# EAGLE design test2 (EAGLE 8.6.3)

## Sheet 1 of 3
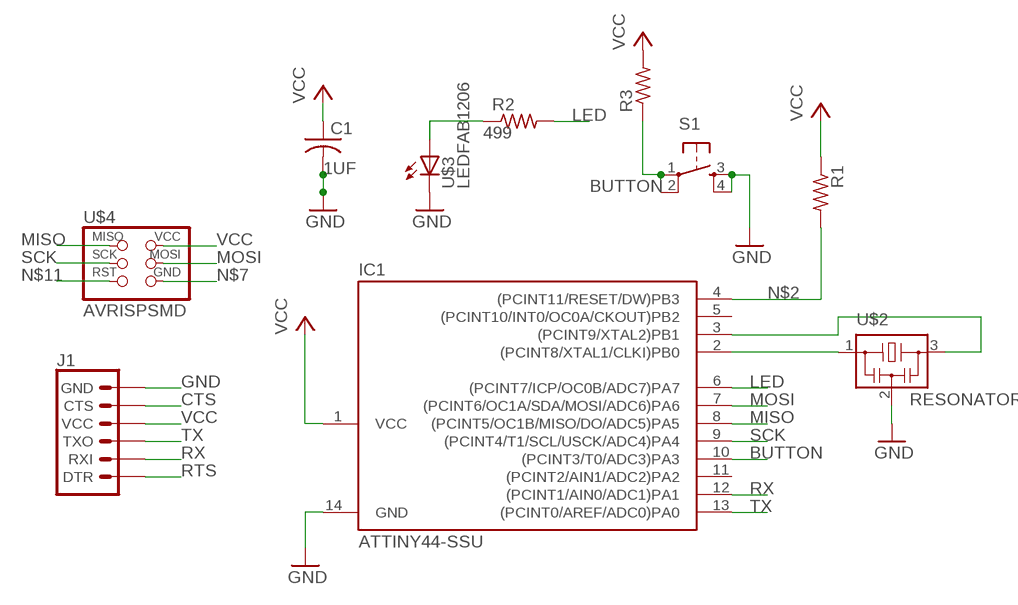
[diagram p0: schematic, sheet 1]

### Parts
C1  C-USC1210  [C1210]
IC1  ATTINY44-SSU  [SOIC14]
J1  6_PIN_SERIAL_TARGETSMD  [1X06-SMD_RA_MALE]
R1  RES-US1206FAB  [R1206FAB]
R2  RES-US1206FAB  [R1206FAB]
R3  RES-US1206FAB  [R1206FAB]
S1  6MM_SWITCH6MM_SWITCH  [6MM_SWITCH]
U$2  RESONATOR  [EFOBM]
U$3  LEDFAB1206  [LED1206FAB]
U$4  AVRISPSMD  [2X03SMD]

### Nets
1UF: C1.2 ; supply symbol labelled GND
499: R2.1 U$3.1(A)
BUTTON: IC1.10((PCINT3/T0/ADC3)PA3) R3.1 S1.1(P) S1.2(P1)
CTS: J1.5(CTS)
GND: J1.6(GND)
LED: IC1.6((PCINT7/ICP/OC0B/ADC7)PA7) R2.2
MISO: IC1.8((PCINT5/OC1B/MISO/DO/ADC5)PA5) U$4.1(MISO)
MOSI: IC1.7((PCINT6/OC1A/SDA/MOSI/ADC6)PA6) U$4.4(MOSI)
N$2: IC1.4((PCINT11/RESET/DW)PB3) R1.2
N$4: IC1.3((PCINT9/XTAL2)PB1) U$2.3
N$7: IC1.14(GND) S1.3(S) S1.4(S1) U$2.2 U$3.2(C) U$4.6(GND) ; supply symbol labelled GND
N$11: U$4.5(RST)
N$23: IC1.2((PCINT8/XTAL1/CLKI)PB0) U$2.1
RTS: J1.1(DTR)
RX: IC1.12((PCINT1/AIN0/ADC1)PA1) J1.2(RXI)
SCK: IC1.9((PCINT4/T1/SCL/USCK/ADC4)PA4) U$4.3(SCK)
TX: IC1.13((PCINT0/AREF/ADC0)PA0) J1.3(TXO)
VCC: C1.1 IC1.1(VCC) J1.4(VCC) R1.1 R3.2 U$4.2(VCC)
Unconnected: IC1.5((PCINT10/INT0/OC0A/CKOUT)PB2) IC1.11((PCINT2/AIN1/ADC2)PA2)

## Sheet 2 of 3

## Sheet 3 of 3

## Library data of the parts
C1 = rcl:C-US: CAPACITOR, American symbol; SPICEPREFIX: C
IC1 = fab:ATTINY44
J1 = SparkFun-Connectors:6_PIN_SERIAL_TARGET: 6-pin header connection for use with the "FTDI BASIC" pinout - TARGET SIDE. Also known as "Arduino Serial Program Header". It is used to mate with our FTDI Basic serial programmers using the Arduino IDE. Note, this device has "TARGET" in the name. It is intended to be used on a design that contains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; PROD_ID: CONN-08971
R1-R3 = fab:RES-US: Resistor (US Symbol)
S1 = fab:6MM_SWITCH: OMRON SWITCH
U$2 = fab:RESONATOR
U$3 = fab:LED: LED
U$4 = fab:AVRISP

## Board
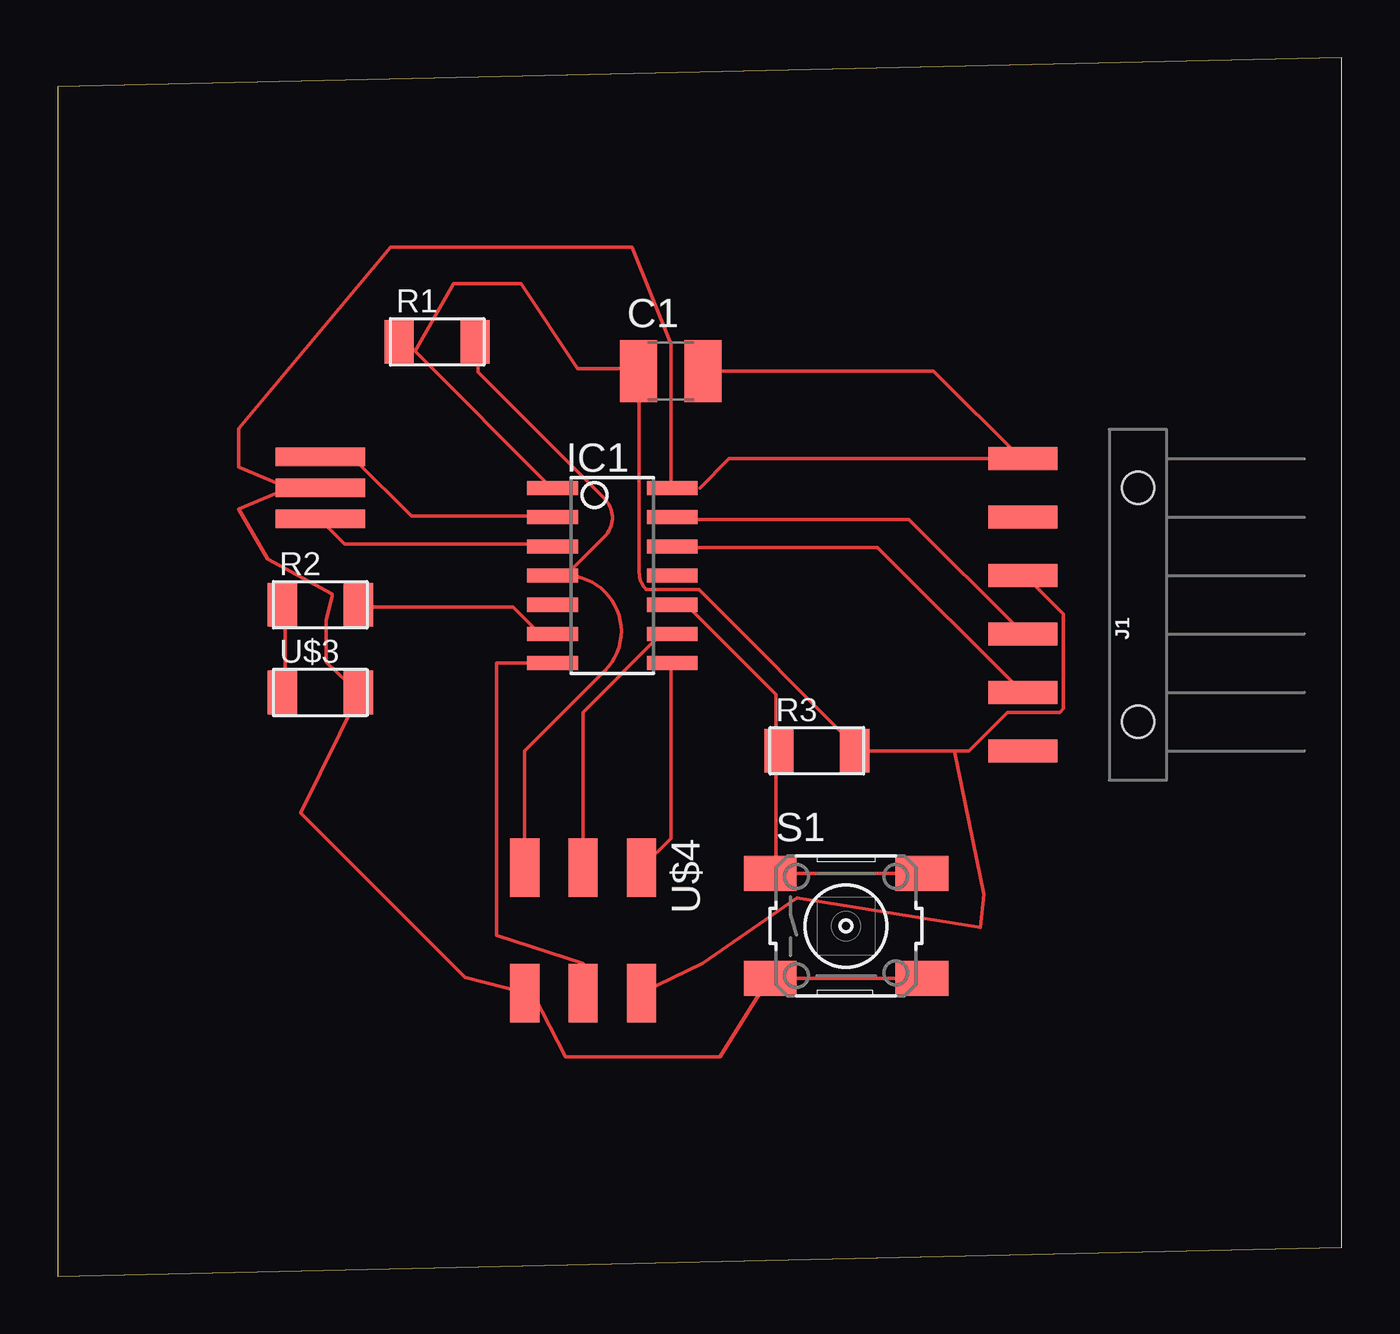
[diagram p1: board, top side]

Size 55.86 x 53.01 mm. Coordinates in mm from the lower left corner, seen from the top.
Outline: 0,0 55.86,1.27 55.86,53.01 0,51.74 0,0
Copper layers (1*16): Top 0.035mm / dielectric 1.5mm / Bottom 0.035mm
Design rules "default": minimum track width 6mil, minimum drill 0.35mm, track to track 6mil, track to pad 6mil, pad to pad 6mil, via to via 6mil, smd to smd 6mil, copper to edge 40mil, drill to drill 6mil, minimum pad ring 10mil, minimum via ring 8mil, stop-mask expansion 4mil, vias tented up to drill 0mil, thermal gap 10mil

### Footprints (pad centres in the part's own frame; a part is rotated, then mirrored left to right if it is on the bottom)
C1210 = smd 1.6 x 2.7: 1 -1.4,0; 2 1.4,0
SOIC14 = smd 0.61 x 2.21: 1 -3.81,-2.603; 2 -2.54,-2.603; 3 -1.27,-2.603; 4 0,-2.603; 5 1.27,-2.603; 6 2.54,-2.603; 7 3.81,-2.603; 8 3.81,2.603; 9 2.54,2.603; 10 1.27,2.603; 11 0,2.603; 12 -1.27,2.603; 13 -2.54,2.603; 14 -3.81,2.603
1X06-SMD_RA_MALE = smd 1 x 3: 1 -6.35,5; 2 -3.81,5; 3 -1.27,5; 4 1.27,5; 5 3.81,5; 6 6.35,5 | hole 1.4: -5.08,0; 5.08,0
R1206FAB = smd 1.27 x 1.905: 1 -1.651,0; 2 1.651,0
6MM_SWITCH = smd 2.286 x 1.524: 1 -3.302,2.286; 2 3.302,2.286; 3 -3.302,-2.286; 4 3.302,-2.286
EFOBM = smd 0.8 x 3.9: 1 -1.35,0; 2 0,0; 3 1.35,0
LED1206FAB = smd 1.27 x 1.905: 1 -1.651,0; 2 1.651,0
2X03SMD = smd 2.54 x 1.27: 1 -2.54,2.54; 2 2.92,2.54; 3 -2.54,0; 4 2.92,0; 5 -2.54,-2.54; 6 2.92,-2.54

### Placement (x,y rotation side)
C1  26.67,39.37 0 top
IC1  24.13,30.48 270 top
J1  46.99,29.21 90 top
R1  16.51,40.64 0 top
R2  11.43,29.21 0 top
R3  33.02,22.86 0 top
S1  34.29,15.24 0 top
U$2  11.43,34.29 270 top
U$3  11.43,25.4 0 top
U$4  22.86,15.24 270 top

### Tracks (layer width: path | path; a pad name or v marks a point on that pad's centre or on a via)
499
  Top 0.152: U$3.1 9.91,25.45 9.91,29.11 R2.1
BUTTON
  Top 0.152: 31.24,22.86 31.24,17.68 31.09,17.53 | 31.24,22.86 31.24,25.3 27.43,29.11 26.82,29.11 IC1.10 | 31.24,22.86 R3.1 | 31.09,17.53 S1.2 | 31.09,17.53 S1.1
LED
  Top 0.152: R2.2 13.11,29.11 19.81,29.11 20.88,28.04 21.49,28.04 IC1.6
MISO
  Top 0.152: U$4.1 26.67,19.05 26.67,26.67 IC1.8
MOSI
  Top 0.152: IC1.7 19.1,26.67 19.1,14.83 22.86,13.61 U$4.4
N$1
  Top 0.152: 27.94,39.37 38.1,39.37 41.91,35.56
N$2
  Top 0.152: 22.1,30.48 arc-135 23.81,26.35 20.32,22.86 20.32,19.05 | 22.1,30.48 23.79,32.17 arc90 23.79,33.82 18.29,39.32 18.29,40.54 R1.2 | IC1.4 21.59,30.48 22.1,30.48
N$3
  Top 0.152: 27.94,34.29 29.21,35.56 40.64,35.56
N$4
  Top 0.152: IC1.3 21.49,31.85 12.5,31.85 11.43,32.92 U$2.3
N$7
  Top 0.152: S1.4 S1.3 30.94,12.95 28.8,9.55 22.1,9.55 20.73,12.19 20.42,12.19 U$4.6 20.27,12.34 17.73,13.01 10.57,20.17 13.11,25.3 U$3.2 11.68,26.72 11.68,28.55 11.94,29.57 11.94,29.67 9.14,31.19 7.87,33.38 10.06,34.29 | 10.06,34.29 7.87,35.2 7.87,36.88 14.48,44.76 24.99,44.76 26.67,40.54 26.67,34.29 IC1.14 | 10.06,34.29 U$2.2
N$23
  Top 0.152: IC1.2 21.49,33.07 15.39,33.07 12.95,35.51 11.43,35.51 U$2.1
RX
  Top 0.152: IC1.12 26.82,31.7 35.66,31.7 41.91,25.45 J1.2
SCK
  Top 0.152: U$4.3 22.86,24.54 26.21,27.89 26.67,27.89 IC1.9
TX
  Top 0.152: IC1.13 26.82,32.92 37.03,32.92 41.91,28.04 J1.3
VCC
  Top 0.152: 15.54,40.23 21.49,34.29 IC1.1 | 15.54,40.23 15.24,40.54 14.94,40.54 R1.1 | 15.54,40.23 17.22,43.18 20.17,43.18 22.61,39.47 25.15,39.47 C1.1 25.3,39.32 25.3,30.61 arc45 25.6,29.87 27.89,29.87 34.9,22.86 | 39.01,22.86 39.62,22.86 41.3,24.54 43.59,24.54 43.74,24.69 43.74,28.8 42.06,30.48 J1.4 | 39.01,22.86 34.9,22.86 | 34.9,22.86 R3.2 34.75,22.86 | 39.01,22.86 40.28,16.61 40.13,15.19 32.16,16.46 28.04,13.61 25.45,12.34 U$4.2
